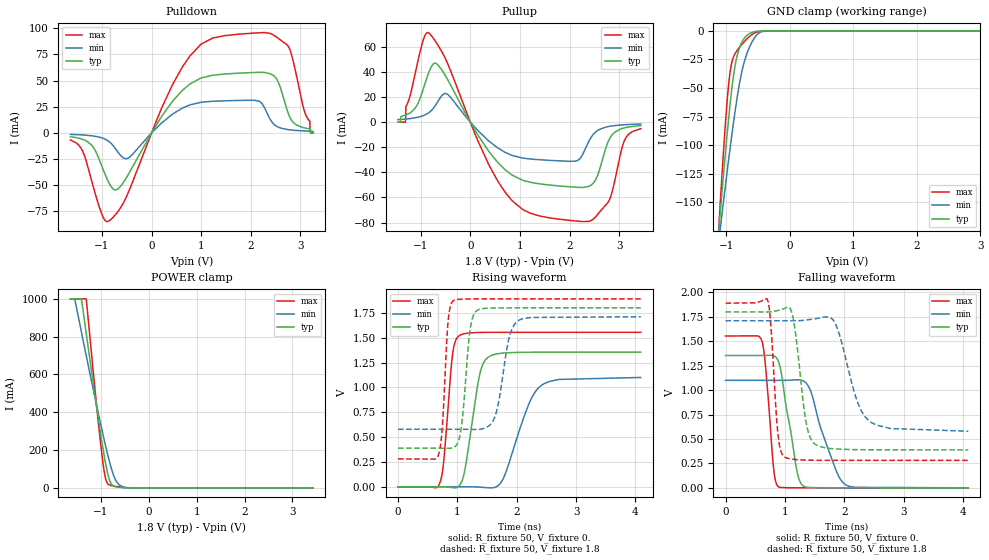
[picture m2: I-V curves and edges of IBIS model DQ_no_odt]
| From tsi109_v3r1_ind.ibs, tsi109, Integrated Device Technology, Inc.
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|   MODEL DQ_no_odt
[Model]   DQ_no_odt
Model_type  I/O
Polarity   Non-Inverting
Enable   Active-Low
|   typ   min   max
|C_comp_off 3.919p 3.933p 3.845p
|C_comp_on 3.698p 3.56p 3.948p
C_comp 3.809p 3.746p 3.896p
Cref  =   20pF
Vmeas =   0.9v
Vinl  =   0.650v
Vinh  =   1.150v
[Model Spec]
[Temperature Range]   25   125   -40
[Voltage Range] 1.8 1.71 1.89
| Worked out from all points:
|   slope of the pulldown table from 0 to 0.27 V, typ, clamps not added: 13.3 ohm
|   slope of the pullup table from 0 to 0.27 V, typ, clamps not added: 15.7 ohm
|   GND clamp passes 1 mA (typ) near -0.57 V on its own axis
|   POWER clamp passes 1 mA (typ) near -0.54 V on its own axis
|   rising waveform, R_fixture 50, V_fixture 0.: 20-80 % time 205ps typ, 380ps min, 124ps max; typ from 0 V to 1.35 V
|   rising waveform, R_fixture 50, V_fixture 1.8: 20-80 % time 121ps typ, 188ps min, 85.6ps max; typ from 0.389 V to 1.8 V
|   falling waveform, R_fixture 50, V_fixture 0.: 20-80 % time 211ps typ, 348ps min, 119ps max; typ from 1.35 V to 0 V
|   falling waveform, R_fixture 50, V_fixture 1.8: 20-80 % time 164ps typ, 316ps min, 100ps max; typ from 1.8 V to 0.389 V
[Pulldown]
-1.636V   -3.649mA   -1.42mA    -6.741mA
-1.394V   -6.111mA   -1.982mA   -17.08mA
-1.215V   -11.4mA    -2.744mA   -44.59mA
-868.9mV  -46.94mA   -7.907mA   -84.38mA
-482.8mV  -40.74mA   -24.38mA   -58.32mA
205.3mV   15.98mA    9.649mA    24.05mA
769.6mV   46.62mA    26.71mA    73.33mA
1.235V    55.1mA     30.21mA    90.62mA
2.235V    57.86mA    27.32mA    95.77mA
2.527V    51.06mA    6.183mA    91.32mA
2.765V    17.53mA    3.042mA    81.91mA
3.26V     0A         0A         0A
[Pullup]
-1.46V    0A         2.056mA    0A
-1.311V   5.643mA    2.505mA    0A
-1.301V   5.791mA    2.542mA    12.38mA
-989.4mV  21.71mA    4.685mA    60.05mA
-840.9mV  39.38mA    7.502mA    71.19mA
-484.4mV  35.79mA    22.74mA    49.06mA
703.7mV   -37.98mA   -24.09mA   -55.96mA
2.263V    -52.03mA   -25.85mA   -79.18mA
2.515V    -46.59mA   -8.159mA   -75.86mA
2.788V    -14.69mA   -3.435mA   -63.09mA
3.105V    -4.545mA   -2.034mA   -14.88mA
3.436V    -2.732mA   -1.461mA   -5.126mA
[GND Clamp]
-1.636V   -543.7mA   -441.2mA   -698mA
-1.118V   -176.6mA   -185.6mA   -175mA
-1.08V    -150.9mA   -167.3mA   -139.5mA
-987.6mV  -92.79mA   -125mA     -64.32mA
-924.6mV  -57.85mA   -97.43mA   -31.77mA
-871.4mV  -34.73mA   -75.48mA   -21.33mA
-813.3mV  -19.18mA   -53.93mA   -16.14mA
-735.9mV  -8.366mA   -31.74mA   -10.82mA
-639mV    -2.666mA   -15.21mA   -5.297mA
-503.5mV  -320uA     -2.798mA   -973.8uA
-305mV    -30.16uA   -47.08uA   -296.9uA
3.26V     0A         0A         0A
[Power Clamp]
-1.636V   1A         1A         1A
-1.549V   1A         1A         1A
-1.411V   1A         828.4mA    1A
-1.308V   819.5mA    701.2mA    1A
-1.067V   389.9mA    409.5mA    378.6mA
-985.5mV  253.4mA    314.2mA    188.6mA
-913.7mV  144.6mA    234mA      62.39mA
-847.1mV  63.87mA    164mA      18.97mA
-780.5mV  20.7mA     101.5mA    12.1mA
-683.2mV  5.068mA    36.78mA    7.528mA
-483.3mV  394.4uA    2.059mA    1.231mA
3.436V    0A         0A         0A
[Ramp]
dV/dt_r .812/205.375p .66/380.602p .932/123.936p
dV/dt_f .847/163.938p .679/315.888p .965/99.968p
[Rising Waveform]
R_fixture = 50
V_fixture = 0.
0s        0V         0V         0V
700ps     244.5uV    -2.152uV   31.55mV
770ps     49.9uV     875.3nV    255.6mV
920ps     -8.207mV   73.82uV    1.334V
1.04ns    16.71mV    185.6uV    1.523V
1.37ns    1.113V     -2.911mV   1.552V
1.51ns    1.299V     -9.011mV   1.553V
1.77ns    1.345V     78.26mV    1.554V
2.43ns    1.354V     1.026V     1.554V
4.09ns    1.354V     1.1V       1.554V
[Rising Waveform]
R_fixture = 50
V_fixture = 1.8
V_fixture_min = 1.71
V_fixture_max = 1.89
0s        388.5mV    578.6mV    281mV
680ps     388.4mV    578.7mV    318.7mV
740ps     388mV      578.7mV    550.7mV
850ps     387.5mV    578.7mV    1.696V
940ps     397.2mV    578.7mV    1.875V
1.05ns    535.1mV    578.4mV    1.886V
1.33ns    1.773V     577.6mV    1.89V
1.63ns    1.798V     701.1mV    1.89V
2.03ns    1.8V       1.672V     1.89V
4.09ns    1.8V       1.71V      1.89V
[Falling Waveform]
R_fixture = 50
V_fixture = 0.
0s        1.354V     1.1V       1.554V
620ps     1.354V     1.1V       1.491V
680ps     1.355V     1.1V       1.208V
820ps     1.349V     1.1V       145.9mV
900ps     1.278V     1.1V       8.41mV
1.2ns     183.3mV    1.105V     710uV
1.31ns    19.37mV    1.094V     400.2uV
1.86ns    480.7uV    183.1mV    21.03uV
2.02ns    258.4uV    33.45mV    9.172uV
4.09ns    0V         23.14uV    0V
[Falling Waveform]
R_fixture = 50
V_fixture = 1.8
V_fixture_min = 1.71
V_fixture_max = 1.89
0s        1.8V       1.71V      1.89V
720ps     1.8V       1.71V      1.903V
880ps     1.815V     1.71V      568.6mV
1ns       1.837V     1.71V      313.4mV
1.13ns    1.762V     1.71V      293.2mV
1.35ns    695.3mV    1.717V     284.2mV
1.51ns    446.5mV    1.73V      282.3mV
1.84ns    399.2mV    1.694V     281.2mV
2.42ns    389.6mV    685.4mV    281mV
4.09ns    388.5mV    579.6mV    281mV
